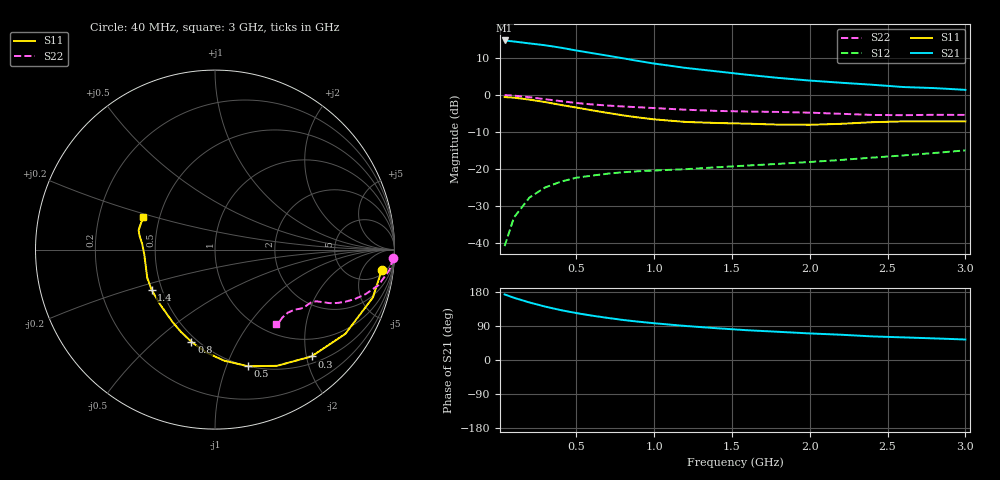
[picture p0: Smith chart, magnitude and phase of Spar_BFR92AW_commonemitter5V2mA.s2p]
! Filename:  BFR92AWA.S2P  Version:  4.0
! NXP part #: BFR92AW  Date: Jun 1994
! Bias condition: Vce=5V, Ic=2mA
#  MHz  S  MA  R  50
! Freq  S11  S21  S12  S22  !GUM [dB]
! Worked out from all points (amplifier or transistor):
!   21 points, 40 MHz to 3 GHz, reference 50 ohm
!   highest |S21| = 14.8 dB at 40 MHz (marker M1)
!   |S21| within 3 dB of that: start of sweep to 541.3 MHz
!   unconditionally stable (mu >= 1): 1.167 GHz to end of sweep
!   at 300 MHz: K = 0.32, MSG = 19.2 dB, |S12| = -25.0 dB
!   at 1 GHz: K = 0.87, MSG = 14.5 dB, |S12| = -20.4 dB
!   at 3 GHz: K = 1.27, MAG = 5.1 dB, |S12| = -15.0 dB
!   S11 on the Smith chart (normalised r, x): 40 MHz: 7, -13; 300 MHz: 0.63, -2.10; 500 MHz: 0.50, -1.20; 800 MHz: 0.47, -0.66; 1.4 GHz: 0.44, -0.24; 3 GHz: 0.41, +0.18
40  0.937 -6.8  5.465 173.1  0.009 85.5  0.995 -2.7
100  0.919 -16.9  5.29 164.2  0.022 78.6  0.979 -6.6
200  0.865 -32.8  4.984 151.8  0.041 69.5  0.933 -12.2
300  0.802 -47.9  4.707 141.0  0.056 61.8  0.876 -16.4
400  0.734 -61.9  4.367 131.7  0.067 56.6  0.826 -19.5
500  0.676 -74.1  3.999 123.9  0.076 53.0  0.78 -21.9
600  0.621 -85.3  3.691 117.1  0.081 50.9  0.745 -23.5
700  0.573 -95.4  3.406 111.2  0.086 49.6  0.72 -24.5
800  0.53 -104.4  3.138 105.7  0.09 49.0  0.699 -25.2
900  0.496 -112.5  2.883 101.1  0.093 48.7  0.682 -25.6
1000  0.468 -120.3  2.663 97.0  0.095 49.0  0.665 -26.1
1200  0.432 -135.3  2.328 89.9  0.099 50.3  0.632 -27.1
1400  0.418 -147.7  2.09 83.9  0.105 52.5  0.609 -29.1
1600  0.409 -157.3  1.875 78.5  0.111 55.3  0.597 -31.6
1800  0.397 -166.1  1.701 74.4  0.117 59.0  0.589 -33.4
2000  0.395 -176.0  1.567 70.1  0.124 62.2  0.577 -34.8
2200  0.407 175.5  1.464 66.7  0.132 65.2  0.556 -37.0
2400  0.428 169.4  1.376 62.3  0.142 67.8  0.537 -40.8
2600  0.439 165.7  1.281 59.7  0.152 70.1  0.533 -45.1
2800  0.438 161.2  1.239 57.0  0.164 72.8  0.539 -48.3
3000  0.438 155.5  1.173 54.1  0.178 74.9  0.537 -50.4
